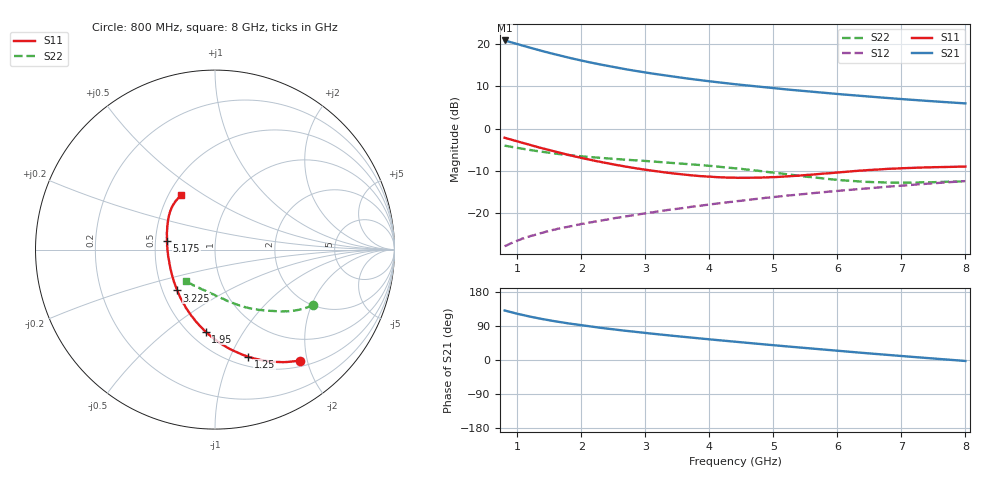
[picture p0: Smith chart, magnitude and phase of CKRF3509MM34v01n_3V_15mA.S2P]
! CHUO DENSHI KOGYO Co.,Ltd.
! 15. August 2018
! CKRF3509MM34_FR4
! N-channel HJ-FETIC
! Vdd = 3 V, Idd = 15.4 mA
# Hz S  MA  R 50
!	f	S11	S21	S12	S22
!	Hz	MAG	ANG	MAG	ANG	MAG	ANG	MAG	ANG
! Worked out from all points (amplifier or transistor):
!   289 points, 800 MHz to 8 GHz, reference 50 ohm
!   highest |S21| = 20.8 dB at 800 MHz (marker M1)
!   |S21| within 3 dB of that: start of sweep to 1.517 GHz
!   unconditionally stable (mu >= 1): 3.412 GHz to end of sweep
!   at 2 GHz: K = 0.82, MSG = 19.2 dB, |S12| = -22.4 dB
!   at 4.4 GHz: K = 1.05, MAG = 12.4 dB, |S12| = -17.2 dB
!   at 8 GHz: K = 1.02, MAG = 8.2 dB, |S12| = -12.4 dB
!   lowest NFmin = 0.29 dB at 1.5 GHz
!   S11 on the Smith chart (normalised r, x): 800 MHz: 0.60, -1.87; 1.25 GHz: 0.60, -1.17; 1.95 GHz: 0.60, -0.69; 3.225 GHz: 0.60, -0.30; 5.175 GHz: 0.57, +0.06; 8 GHz: 0.58, +0.40
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8e8  0.7787 -52.6  10.91 130.7  0.04114 65.0  0.6289 -29.4
9e8  0.7422 -57.5  10.39 126.2  0.04454 62.9  0.6096 -31.7
1e9  0.7065 -62.2  9.88 121.9  0.0479 61.4  0.5918 -33.8
1.125e9  0.6645 -67.7  9.29 117.1  0.05168 59.5  0.5703 -36.2
1.25e9  0.6256 -72.7  8.747 112.6  0.05506 58.1  0.5506 -38.3
1.4e9  0.5824 -78.4  8.145 107.7  0.05951 56.5  0.5303 -40.4
1.575e9  0.538 -84.6  7.527 102.5  0.06437 55.1  0.5094 -42.5
1.75e9  0.4993 -90.3  6.989 97.8  0.06863 54.1  0.4922 -44.3
1.95e9  0.4602 -96.5  6.452 92.8  0.07375 52.8  0.4745 -46.1
2e9  0.4513 -98.1  6.327 91.6  0.07553 52.9  0.4717 -46.5
2.25e9  0.4109 -105.4  5.776 86.0  0.08118 51.7  0.4543 -48.6
2.55e9  0.3722 -113.8  5.226 79.8  0.08878 50.2  0.4368 -50.7
2.9e9  0.3366 -123.6  4.708 73.2  0.09777 48.9  0.4191 -53.3
3.2e9  0.3118 -132.0  4.341 67.8  0.1057 47.4  0.4043 -55.4
3.225e9  0.3102 -132.8  4.312 67.4  0.1064 47.3  0.4032 -55.6
3.775e9  0.279 -148.8  3.786 58.1  0.1211 44.4  0.3765 -60.1
4.4e9  0.2637 -167.7  3.329 48.2  0.1384 40.9  0.3401 -66.2
5.175e9  0.2725 169.9  2.908 36.5  0.1605 35.7  0.292 -76.8
5.6e9  0.2863 158.8  2.714 30.2  0.1729 32.7  0.2669 -84.7
6.15e9  0.3101 147.1  2.5 22.2  0.1885 28.6  0.2436 -96.2
6.8e9  0.3355 136.5  2.285 13.2  0.2071 23.5  0.2321 -111.0
8e9  0.3569 121.9  1.979 -2.6  0.2402 13.9  0.2395 -132.5
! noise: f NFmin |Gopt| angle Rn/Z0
1.5e+09  0.29  0.436  33.5  0.11
1.7e+09  0.31  0.411  36  0.11
1.9e+09  0.32  0.386  39.6  0.11
2.1e+09  0.34  0.361  42.8  0.11
2.3e+09  0.36  0.335  46.4  0.11
2.6e+09  0.4  0.306  55.5  0.1
2.8e+09  0.41  0.28  60.5  0.09
3e+09  0.43  0.252  65  0.1
3.2e+09  0.44  0.228  73  0.09
3.5e+09  0.47  0.205  85  0.09
